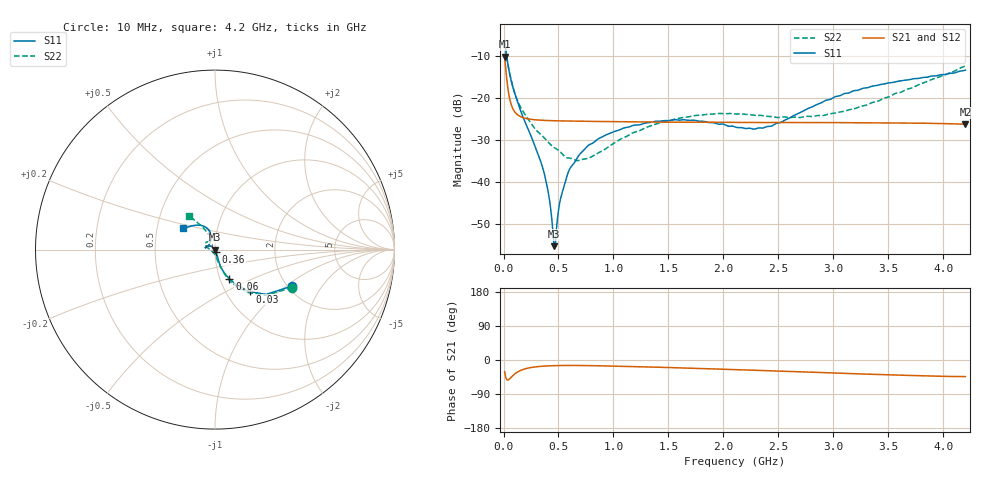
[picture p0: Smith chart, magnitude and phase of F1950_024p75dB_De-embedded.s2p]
! Integrated Device Technology
! Corporate Headquarters
! 6024 Silver Creek Valley Road
! San Jose, CA 95138  USA
! Phone:  1-408-284-8200
! Toll Free:  1-800-223-1366
! Webpage:  http://www.idt.com/
! Timing and RF Division
! 515 Groton Road, Suite 102
! Westford, MA 01886-6024
! Device:  F1950
! Description: 7-bit 0.25 dB Digital Step Attenuator
! Frequency:  150.0 -  4000.00 MHz
! Package:  4x4 mm Thin QFN Plastic Package: 24 pin
! Ports:  2 RF, 12 DC
!  Pin  1  = D0
!  Pin  2  = VDD
!  Pin  3  = Vmode
!  Pin  4  = GND
!  Pin  5  = RF1  =  Port 1
!  Pin  6  = GND
!  Pin  7  = GND
!  Pin  8  = GND
!  Pin  9  = GND
!  Pin 10  = GND
!  Pin 11  = GND
!  Pin 12  = GND
!  Pin 13  = GND
!  Pin 14  = RF2  =  Port 2
!  Pin 15  = GND
!  Pin 16  = LE
!  Pin 17  = CLK
!  Pin 18  = DATE
!  Pin 19  = D6
!  Pin 20  = D5
!  Pin 21  = D4
!  Pin 22  = D3
!  Pin 23  = D2
!  Pin 24  = D1
! State:  99
! Atten State:  24.75 dB
! Voltage:  +5.00 Volts
! Current:  Not Measured mA
! Data:  The device was measured on a the F195X evaluation board which has
!  individual transmission lines to the RF pins.  Data was collected
!  using a calibrated network analyzer.  The evaluation board was
!  de-embedded using a TRL calibration technique.
!  The reference plane is the edge of the package pin.
! Misc:  Board 2019
!  Action Tracker AT0250
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# GHz S dB R 50
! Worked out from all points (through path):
!   420 points, 10 MHz to 4.2 GHz, reference 50 ohm
!   highest |S21| = -10.25 dB at 10 MHz (marker M1); lowest = -26.3 dB at 4.2 GHz (marker M2)
!   group delay of S21, straight-line fit = 18.1 ps
!   lowest |S11| = -55.3 dB at 460 MHz (marker M3), VSWR 1.00, Z = 49.9 - j0.124 ohm
!   |S11| at or under -10 dB: 28.06 MHz to end of sweep
!   |S22| runs from -35.0 to -6.4 dB; largest |S21 - S12| = 0.00011
!   S11 on the Smith chart (normalised r, x): 10 MHz: 2.12, -1.11; 30 MHz: 1.29, -0.66; 60 MHz: 1.11, -0.37; 360 MHz: 1.01, -0.03; 4.2 GHz: 0.68, +0.17
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0.01  -6.44 -25.2  -10.25 -30.8  -10.25 -30.8  -6.38 -26.2
0.03  -10.38 -50.4  -15.68 -52.0  -15.68 -52.0  -10.31 -51.9
0.06  -14.87 -63.7  -20.67 -48.6  -20.68 -48.6  -14.65 -65.2
0.1  -18.76 -70.4  -23.28 -37.4  -23.28 -37.3  -18.74 -70.7
0.15  -22.70 -72.3  -24.43 -28.3  -24.43 -28.3  -22.00 -74.9
0.36  -37.03 -69.5  -25.38 -16.2  -25.38 -16.2  -29.26 -85.4
0.41  -42.98 -76.7  -25.44 -15.4  -25.44 -15.4  -30.65 -87.6
0.45  -52.20 -103.8  -25.48 -15.0  -25.48 -15.0  -31.68 -93.1
0.46  -55.32 -133.6  -25.48 -14.9  -25.49 -14.9  -31.87 -94.8
0.48  -51.73 160.2  -25.50 -14.8  -25.50 -14.8  -32.18 -97.7
0.52  -43.90 142.3  -25.52 -14.5  -25.52 -14.5  -32.96 -101.1
0.58  -38.41 136.0  -25.55 -14.4  -25.55 -14.4  -34.31 -113.1
0.71  -33.01 138.6  -25.60 -14.5  -25.60 -14.6  -34.72 -138.1
0.99  -28.23 147.9  -25.70 -16.0  -25.70 -16.0  -31.06 -179.0
1.41  -25.59 163.5  -25.79 -19.1  -25.79 -19.1  -26.08 161.1
1.73  -25.35 169.0  -25.83 -21.7  -25.82 -21.7  -24.28 152.6
2.11  -26.99 158.8  -25.87 -25.5  -25.87 -25.5  -23.86 142.9
2.43  -26.79 127.3  -25.89 -28.3  -25.89 -28.3  -24.46 132.2
2.81  -22.13 106.0  -25.91 -32.3  -25.91 -32.4  -24.45 116.9
3.19  -18.32 109.1  -25.95 -36.2  -25.94 -36.2  -22.61 111.2
3.51  -16.45 117.8  -25.98 -39.2  -25.98 -39.2  -19.73 113.9
4.2  -13.44 145.9  -26.29 -43.8  -26.28 -43.9  -12.44 127.4
